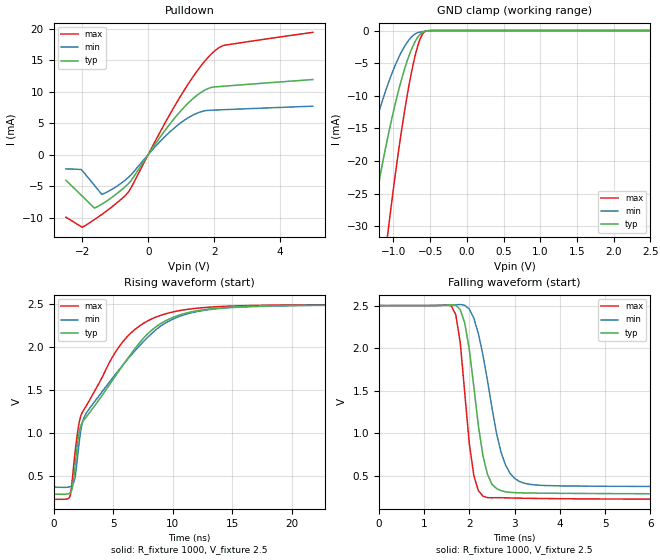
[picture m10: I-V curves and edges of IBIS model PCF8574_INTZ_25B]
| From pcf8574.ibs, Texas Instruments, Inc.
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[Model]   PCF8574_INTZ_25B
Model_type  Open_drain
Enable   Active-Low
Vref =   2.5
Rref =   4700
Cref =   10p
Vmeas =   1.25
| variable   typ   min   max
C_comp   0.80pF   0.75pF   0.89pF
| C_pulldown   0.79pF   0.73pF   0.85pF
| C_tri-state   0.80pF   0.75pF   0.89pF
[Temperature Range]   40   100   -40
| Ambient temperature   25   85   -40
[Voltage range]   2.5   2.5   2.5
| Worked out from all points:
|   slope of the pulldown table from 0 to 0.375 V, typ, clamps not added: 131 ohm
|   GND clamp passes 1 mA (typ) near -0.67 V on its own axis
|   rising waveform, R_fixture 1000, V_fixture 2.5: 20-80 % time 5.36ns typ, 5.51ns min, 3.97ns max; typ from 0.287 V to 2.5 V
|   falling waveform, R_fixture 1000, V_fixture 2.5: 20-80 % time 329ps typ, 454ps min, 249ps max; typ from 2.5 V to 0.287 V
[GND Clamp]
| PCF8574_INTZ_25B
|   Voltage   I(typ)   I(min)   I(max)
-2.5V     -133mA     -90.53mA   -210.3mA
-1.59V    -50.07mA   -31.23mA   -86.94mA
-1.56V    -47.82mA   -29.5mA    -83.34mA
-1.315V   -30.65mA   -17.09mA   -55.3mA
-1.085V   -16.81mA   -8.563mA   -31.92mA
-1.06V    -15.47mA   -7.773mA   -29.61mA
-945mV    -9.85mA    -4.548mA   -19.67mA
-840mV    -5.601mA   -2.28mA    -11.78mA
-690mV    -1.405mA   -430.4uA   -3.231mA
-605mV    -289.1uA   -175.4uA   -571.8uA
-520mV    -43.98uA   -43.05uA   -12.59uA
2.5V      258.1pA    411pA      63.41pA
[Pulldown]
| PCF8574_INTZ_25B
|   Voltage   I(typ)   I(min)   I(max)
-2.5V     -4.083mA   -2.27mA    -9.942mA
-2.005V   -6.587mA   -2.537mA   -11.53mA
-1.635V   -8.485mA   -4.874mA   -10.33mA
-1.415V   -7.894mA   -6.292mA   -9.53mA
-1.37V    -7.75mA    -6.249mA   -9.36mA
-575mV    -4.467mA   -3.495mA   -5.736mA
370mV     2.828mA    2.134mA    3.669mA
1.035V    7.208mA    5.228mA    9.732mA
1.615V    9.919mA    6.822mA    14.18mA
2.085V    10.78mA    7.087mA    16.75mA
2.335V    10.88mA    7.142mA    17.39mA
5V        11.92mA    7.692mA    19.42mA
[Ramp]
| PCF8574_INTZ_25B
| variable   typ   min   max
dV/dt_r   1.33/5.36E-09   1.28/5.51E-09   1.36/3.97E-09
dV/dt_f   1.33/3.31E-10   1.29/4.60E-10   1.37/2.52E-10
R_load = 1000
[Rising Waveform]
| PCF8574_INTZ_25B
R_fixture =   1000
C_fixture =   0
L_fixture =   0
V_fixture =   2.5
V_fixture_min = 2.5
V_fixture_max = 2.5
|   Time   V(typ)   V(min)   V(max)
0s        286.9mV    369.4mV    227.1mV
1.4ns     303.8mV    375.1mV    268.6mV
1.6ns     371.7mV    398.4mV    491mV
1.8ns     609.9mV    475.6mV    765.8mV
2.3ns     1.09V      1.04V      1.204V
2.8ns     1.198V     1.244V     1.33V
5.9ns     1.807V     1.808V     2.079V
9ns       2.278V     2.249V     2.374V
13.4ns    2.452V     2.446V     2.472V
269.9ns   2.5V       2.5V       2.5V
[Falling Waveform]
| PCF8574_INTZ_25B
R_fixture =   1000
C_fixture =   0
L_fixture =   0
V_fixture =   2.5
V_fixture_min = 2.5
V_fixture_max = 2.5
|   Time   V(typ)   V(min)   V(max)
0s        2.5V       2.5V       2.5V
1.6ns     2.509V     2.505V     2.499V
1.8ns     2.453V     2.513V     2.065V
2.1ns     1.548V     2.353V     505.2mV
2.3ns     741.1mV    1.923V     264.8mV
2.5ns     404.1mV    1.302V     245mV
2.7ns     328.5mV    780.5mV    246.2mV
3ns       305.6mV    473.4mV    242mV
4.6ns     295.7mV    381.7mV    232.4mV
269.9ns   286.9mV    369.4mV    227.1mV
